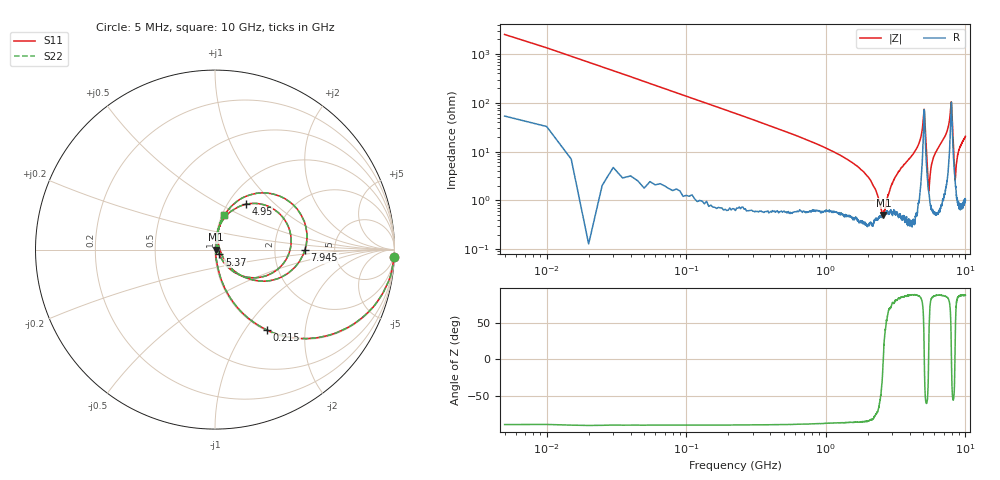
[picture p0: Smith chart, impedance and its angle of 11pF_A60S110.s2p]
! Amotech Co.,Ltd.
! http://www.amotech.co.kr/
! Part Number: A60S110
! These Parameters are Measured in Series Mode Connection
! Operation Temp=25[degC], DC Bias Voltage=0[V]
! Freq. Start=5[MHz] Stop=10[GHz], 2000[Steps]
! Date: Monday, July 13, 2020, 01:35:40
# GHZ S RI R 50.000000
!Freq.(Hz) S11(Real) S11(Imag) S21(Real) S21(Imag) S12(Real) S12(Imag) S22(Real) S22(Imag)
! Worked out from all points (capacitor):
!   2000 points, 5 MHz to 10 GHz, reference 50 ohm
!   read as one part in series: C = 11.6 pF near 55 MHz
!   lowest |Z| = 505 mohm at 2.585 GHz (marker M1)
!   series resonance near 2.581 GHz, so ESL is about 330 pH
!   S11 on the Smith chart (normalised r, x): 5 MHz: 2, -50; 215 MHz: 1.01, -1.27; 4.95 GHz: 1.21, +0.67; 5.37 GHz: 1.05, -0.06; 7.945 GHz: 3.01, -0.01; 10 GHz: 1.02, +0.41
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0.005  0.9976 -0.0395  0.00241 0.0395  0.00241 0.0395  0.9976 -0.0395
0.085  0.7199 -0.4438  0.2801 0.4438  0.2801 0.4438  0.7199 -0.4438
0.215  0.2905 -0.4487  0.7095 0.4487  0.7095 0.4487  0.2905 -0.4487
0.555  0.0581 -0.223  0.9419 0.223  0.9419 0.223  0.0581 -0.223
1.675  0.00676 -0.0498  0.9932 0.0498  0.9932 0.0498  0.00676 -0.0498
2.585  0.00502 0.000218  0.995 -0.000218  0.995 -0.000218  0.00502 0.000218
3.34  0.00636 0.0389  0.9936 -0.0389  0.9936 -0.0389  0.00636 0.0389
4.545  0.0217 0.1225  0.9783 -0.1225  0.9783 -0.1225  0.0217 0.1225
4.95  0.1706 0.2524  0.8294 -0.2524  0.8294 -0.2524  0.1706 0.2524
5.005  0.2934 0.2429  0.7066 -0.2429  0.7066 -0.2429  0.2934 0.2429
5.145  0.2239 -0.1569  0.7761 0.1569  0.7761 0.1569  0.2239 -0.1569
5.37  0.0241 -0.0267  0.9759 0.0267  0.9759 0.0267  0.0241 -0.0267
5.475  0.0143 0.00688  0.9857 -0.00688  0.9857 -0.00688  0.0143 0.00688
5.79  0.00966 0.0607  0.9903 -0.0607  0.9903 -0.0607  0.00966 0.0607
6.67  0.028 0.1416  0.972 -0.1416  0.972 -0.1416  0.028 0.1416
7.755  0.2786 0.3161  0.7214 -0.3161  0.7214 -0.3161  0.2786 0.3161
7.945  0.5012 -0.00102  0.4988 0.00102  0.4988 0.00102  0.5012 -0.00102
8.06  0.2635 -0.1759  0.7365 0.1759  0.7365 0.1759  0.2635 -0.1759
8.335  0.0388 -0.031  0.9612 0.031  0.9612 0.031  0.0388 -0.031
8.455  0.0228 0.0128  0.9772 -0.0128  0.9772 -0.0128  0.0228 0.0128
8.94  0.0188 0.1003  0.9812 -0.1003  0.9812 -0.1003  0.0188 0.1003
10  0.0495 0.1934  0.9505 -0.1934  0.9505 -0.1934  0.0495 0.1934
